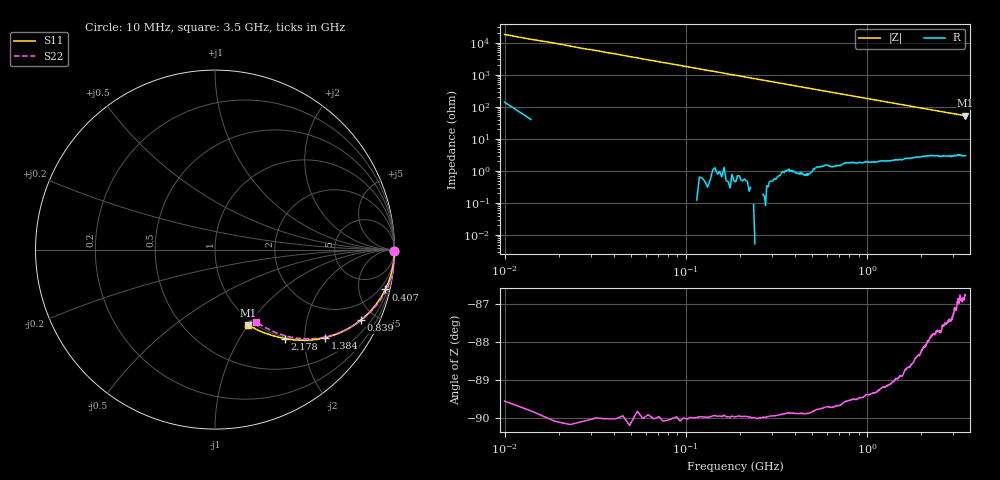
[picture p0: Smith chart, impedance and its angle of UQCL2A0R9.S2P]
! AVX Corporation
! Date:  10/27/06
! Part No:  UQCL2A0R9
! Description:  Ultra Low ESR Microwave capacitors
! Mounting Orientation:  Horizontal
# GHZ S DB R 50
! Freq  |S11|  S11 Ph  |S21|  S21 Ph  |S12|  S12 Ph  |S22|  S22 Ph
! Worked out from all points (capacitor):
!   801 points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, 10 MHz to 3.5 GHz, reference 50 ohm
!   read as one part in series: C = 876 fF near 27 MHz
!   lowest |Z| = 52.8 ohm at 3.5 GHz (marker M1)
!   S11 on the Smith chart (normalised r, x): 10 MHz: open; 407 MHz: 0.95, -8.56; 839 MHz: 0.98, -4.15; 1.384 GHz: 0.98, -2.52; 2.178 GHz: 0.97, -1.60; 3.5 GHz: 0.94, -1.00
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0.01  -0.01 -0.3  -45.16 89.2  -45.27 88.5  -0.01 -0.5
0.019  -0.01 -0.7  -39.74 89.5  -39.70 89.5  -0.01 -0.6
0.036  -0.01 -1.2  -34.01 88.8  -33.97 88.8  -0.01 -1.2
0.049  -0.01 -1.7  -31.36 88.6  -31.31 88.5  -0.01 -1.5
0.062  -0.01 -2.1  -29.29 87.9  -29.24 87.9  -0.01 -2.0
0.075  -0.01 -2.5  -27.65 87.6  -27.61 87.6  -0.01 -2.4
0.097  -0.01 -3.2  -25.44 86.8  -25.40 86.9  -0.01 -3.1
0.123  -0.02 -4.1  -23.37 86.0  -23.33 85.9  -0.01 -4.0
0.171  -0.04 -5.6  -20.54 84.4  -20.50 84.4  -0.01 -5.5
0.232  -0.08 -7.6  -17.93 82.5  -17.88 82.4  -0.03 -7.5
0.315  -0.13 -10.2  -15.33 79.8  -15.28 79.8  -0.08 -10.1
0.407  -0.22 -13.2  -13.20 76.8  -13.15 76.8  -0.17 -12.9
0.494  -0.32 -15.8  -11.61 74.1  -11.56 74.1  -0.27 -15.6
0.595  -0.47 -18.9  -10.14 71.0  -10.09 70.9  -0.41 -18.6
0.839  -0.89 -25.8  -7.58 63.9  -7.54 63.8  -0.85 -25.4
1.175  -1.60 -34.2  -5.39 55.4  -5.34 55.3  -1.57 -33.6
1.384  -2.09 -38.7  -4.48 50.8  -4.43 50.7  -2.07 -38.0
1.755  -3.00 -45.5  -3.37 43.8  -3.34 43.7  -2.98 -44.5
2.178  -4.00 -51.8  -2.61 37.6  -2.58 37.6  -4.00 -50.0
2.34  -4.37 -53.9  -2.40 35.6  -2.36 35.6  -4.38 -51.8
2.92  -5.59 -60.5  -1.88 30.1  -1.84 30.0  -5.62 -56.8
3.5  -6.73 -66.2  -1.59 25.7  -1.53 25.8  -6.73 -60.4
